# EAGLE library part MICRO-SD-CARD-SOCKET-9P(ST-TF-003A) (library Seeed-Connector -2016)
320090000
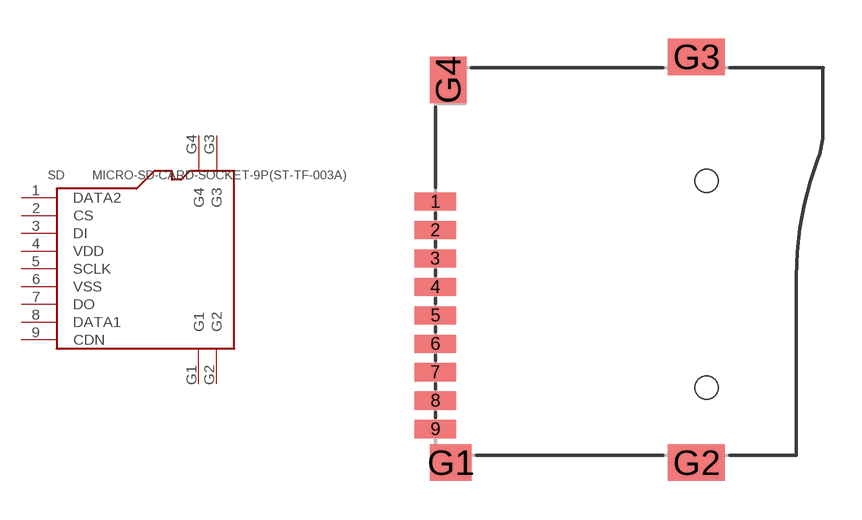
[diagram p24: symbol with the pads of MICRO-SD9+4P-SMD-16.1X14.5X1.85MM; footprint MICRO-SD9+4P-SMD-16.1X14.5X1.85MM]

Designator prefix SD

## MICRO-SD-CARD-SOCKET-9P(ST-TF-003A) (MPN: ST-TF-003A; VALUE: ST-TF-003A)  [MICRO-SD9+4P-SMD-16.1X14.5X1.85MM]
1  DATA2
2  CS
3  DI
4  VDD
5  SCLK
6  VSS
7  DO
8  DATA1
9  CDN
G1  G1
G2  G2
G3  G3
G4  G4

## Footprint MICRO-SD9+4P-SMD-16.1X14.5X1.85MM (pad centres in mm)
smd 1.6 x 0.7: 1 0,2.25; 2 0,1.15; 3 0,0.05; 4 0,-1.05; 5 0,-2.15; 6 0,-3.25; 7 0,-4.35; 8 0,-5.45; 9 0,-6.55
smd 1.6 x 1.4: G1 0.6,-7.85
smd 2.2 x 1.4: G2 10.1,-7.85; G3 10.1,7.85
smd 1.4 x 1.8: G4 0.5,6.95
hole 0.9 at 10.5,-4.95
hole 0.9 at 10.5,3.05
